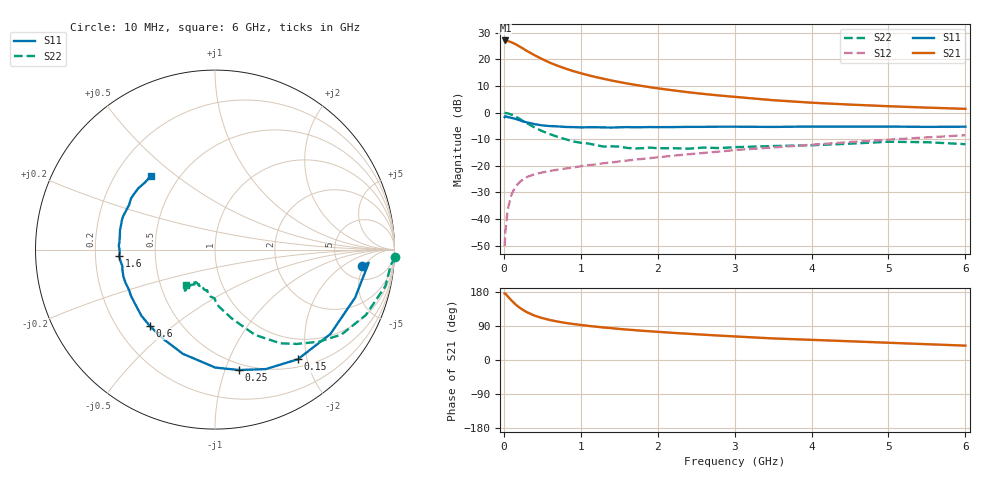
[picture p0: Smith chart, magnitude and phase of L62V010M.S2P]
!  INFINEON TECHNOLOGIES Small Signal Semiconductors
! BFR380L3 , Si-NPN RF-Transistor in TSLP-3-1
!  Vce=2 V,  Ic=10 mA
! Common Emitter S-Parameters:  07. March 2005
#  GHz  S  MA  R  50
! f  S11  S21  S12  S22
! GHz  Mag  Ang  Mag  Ang  Mag  Ang  Mag  Ang
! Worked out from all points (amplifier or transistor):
!   36 points, 10 MHz to 6 GHz, reference 50 ohm
!   highest |S21| = 27.1 dB at 20 MHz (marker M1)
!   |S21| within 3 dB of that: start of sweep to 247.3 MHz
!   unconditionally stable (mu >= 1): 2.178 GHz to 4.815 GHz
!   at 250 MHz: K = 0.26, MSG = 24.6 dB, |S12| = -25.1 dB
!   at 1.4 GHz: K = 0.89, MSG = 15.4 dB, |S12| = -18.7 dB
!   at 6 GHz: K = 0.97, MSG = 5.0 dB, |S12| = -8.5 dB
!   S11 on the Smith chart (normalised r, x): 10 MHz: 7.93, -4.42; 150 MHz: 0.62, -1.84; 250 MHz: 0.44, -1.12; 600 MHz: 0.34, -0.42; 1.6 GHz: 0.30, -0.03; 6 GHz: 0.35, +0.41
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0.01  0.8249 -6.2  22.66 175.8  0.0031 84.7  1.005 -2.4
0.02  0.8596 -4.9  22.71 175.4  0.0058 87.4  0.9833 -5.0
0.05  0.8254 -18.9  22.19 168.0  0.015 80.5  0.9709 -12.1
0.1  0.7966 -36.2  20.95 157.1  0.0291 73.3  0.9159 -23.5
0.15  0.7658 -52.9  19.41 147.1  0.0401 65.5  0.8488 -33.9
0.2  0.7236 -66.9  17.65 138.7  0.0489 60.1  0.7733 -41.6
0.25  0.6843 -78.7  16 132.1  0.0558 55.5  0.6956 -49.1
0.3  0.6571 -89.9  14.43 126.1  0.0618 52.1  0.6364 -55.1
0.4  0.6077 -107.1  11.98 117.0  0.0697 48.6  0.5257 -64.8
0.5  0.5753 -120.0  10.11 110.6  0.0751 46.9  0.4487 -70.6
0.6  0.5593 -130.4  8.659 105.4  0.0805 46.1  0.394 -76.4
0.7  0.5515 -138.0  7.591 101.4  0.0848 46.6  0.3504 -81.3
0.8  0.5389 -145.2  6.742 97.9  0.0891 47.0  0.3175 -86.2
0.9  0.5344 -151.2  6.042 95.0  0.093 47.6  0.2877 -89.4
1.1  0.5318 -159.8  5.036 90.0  0.1028 49.6  0.2632 -95.3
1.4  0.5245 -169.9  4.015 84.0  0.1158 51.9  0.2327 -101.9
1.6  0.5349 -176.2  3.539 80.3  0.1256 53.1  0.2177 -109.3
2.2  0.5355 172.0  2.624 71.6  0.1552 56.6  0.2149 -114.6
3.5  0.5395 152.6  1.713 56.9  0.222 59.0  0.2358 -123.8
4.5  0.5473 145.3  1.416 49.4  0.28 59.6  0.2615 -125.4
5.5  0.5405 136.5  1.243 41.7  0.343 57.5  0.2783 -127.0
6  0.5444 131.0  1.179 37.9  0.3759 56.0  0.2557 -129.1
